(* Logix 5000 AddOnInstructionDefinition export Banner_Q2X_Param_v4; software revision 33.00; part 3 of 3 *)
(* tags used below, declared in another part *)
   Q2X : Banner_Q2X_v4;
   Port_Data : Banner_IOL_Port_v4;
   Port : DINT;
   Local_Control : DINT;
   Command_Being_Processed : BOOL;
   Update_Archive : BOOL;
   Index_Write_Inprocess : INT;
   Inprocess_Index : DINT;
(* Banner_Q2X_Param_v4, continued *)

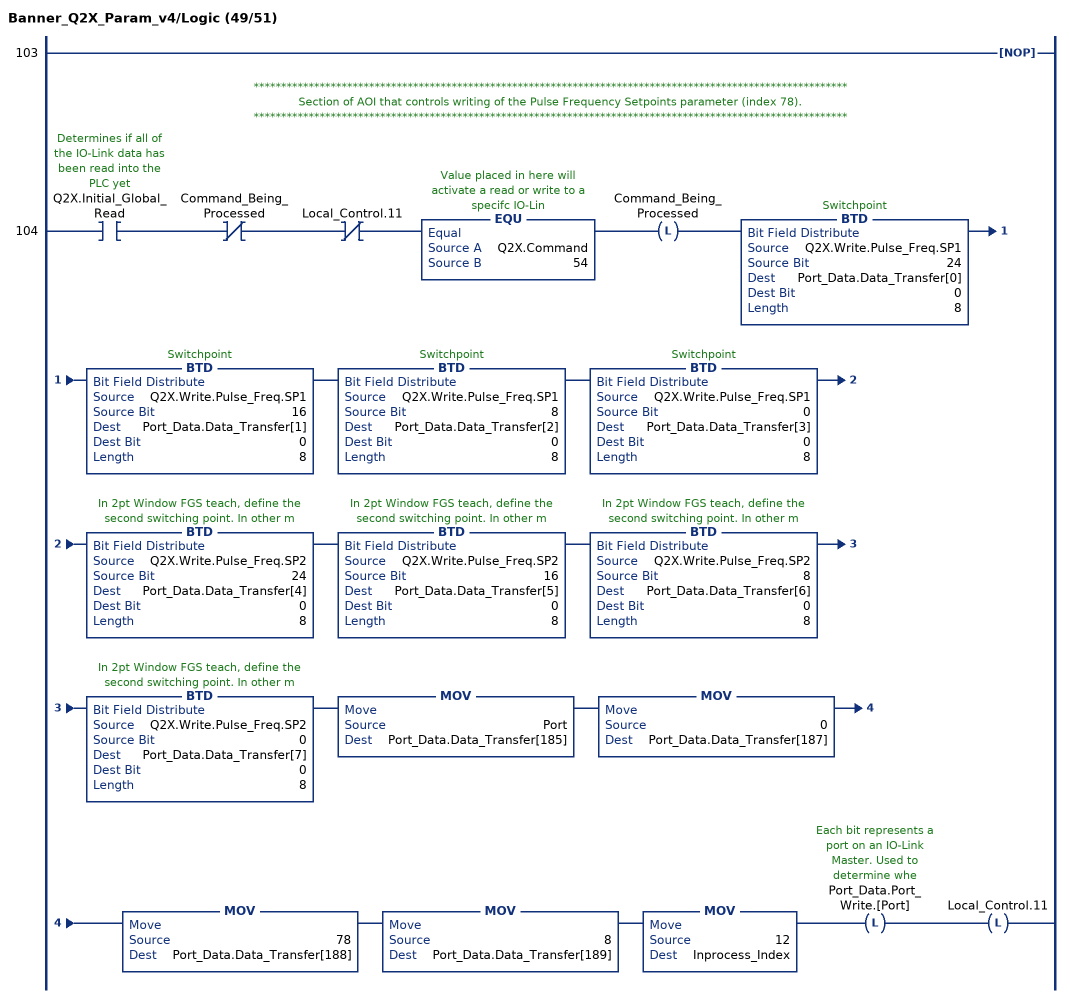
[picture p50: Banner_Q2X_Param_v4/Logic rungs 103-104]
   103: NOP();
   // ************************************************************************************************************
   // Section of AOI that controls writing of the Pulse Frequency Setpoints parameter (index 78).
   // ************************************************************************************************************
   104: XIC(Q2X.Initial_Global_Read)XIO(Command_Being_Processed)XIO(Local_Control.11)EQU(Q2X.Command,54)OTL(Command_Being_Processed)BTD(Q2X.Write.Pulse_Freq.SP1,24,Port_Data.Data_Transfer[0],0,8)BTD(Q2X.Write.Pulse_Freq.SP1,16,Port_Data.Data_Transfer[1],0,8)BTD(Q2X.Write.Pulse_Freq.SP1,8,Port_Data.Data_Transfer[2],0,8)BTD(Q2X.Write.Pulse_Freq.SP1,0,Port_Data.Data_Transfer[3],0,8)BTD(Q2X.Write.Pulse_Freq.SP2,24,Port_Data.Data_Transfer[4],0,8)BTD(Q2X.Write.Pulse_Freq.SP2,16,Port_Data.Data_Transfer[5],0,8)BTD(Q2X.Write.Pulse_Freq.SP2,8,Port_Data.Data_Transfer[6],0,8)BTD(Q2X.Write.Pulse_Freq.SP2,0,Port_Data.Data_Transfer[7],0,8)MOV(Port,Port_Data.Data_Transfer[185])MOV(0,Port_Data.Data_Transfer[187])MOV(78,Port_Data.Data_Transfer[188])MOV(8,Port_Data.Data_Transfer[189])MOV(12,Inprocess_Index)OTL(Port_Data.Port_Write.[Port])OTL(Local_Control.11);
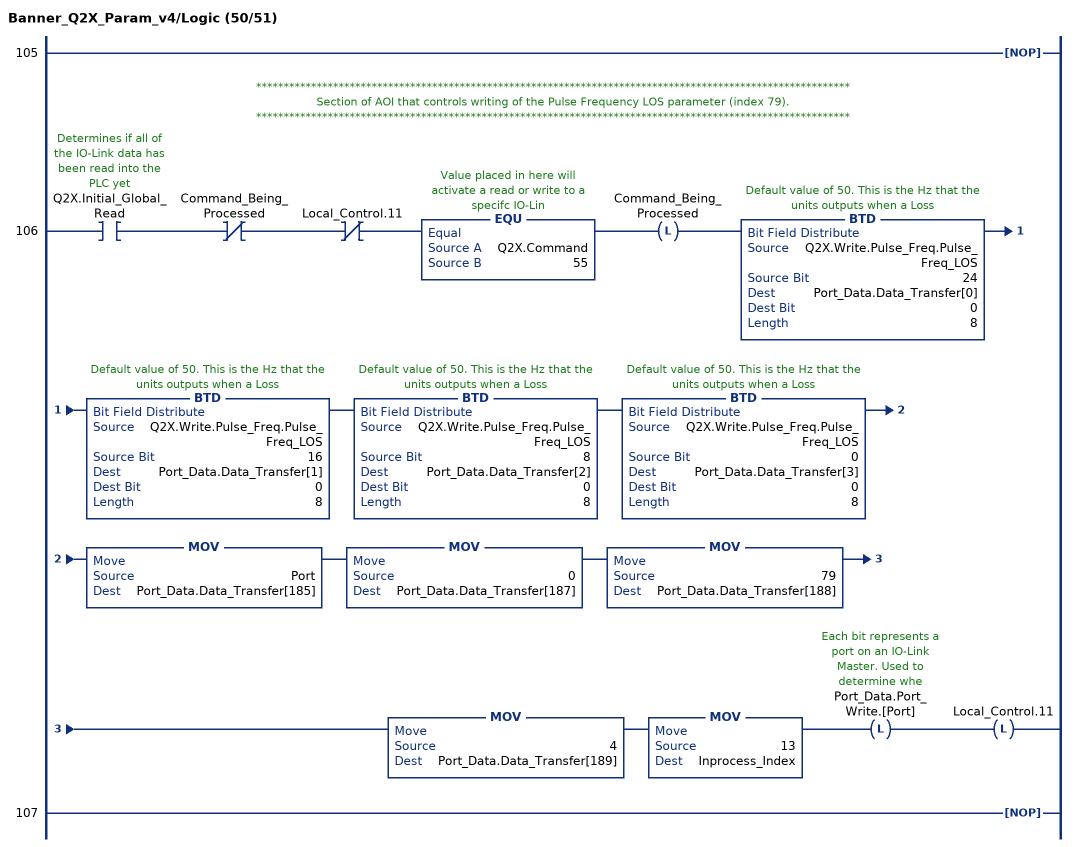
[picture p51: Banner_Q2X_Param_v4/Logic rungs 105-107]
   105: NOP();
   // ************************************************************************************************************
   // Section of AOI that controls writing of the Pulse Frequency LOS parameter (index 79).
   // ************************************************************************************************************
   106: XIC(Q2X.Initial_Global_Read)XIO(Command_Being_Processed)XIO(Local_Control.11)EQU(Q2X.Command,55)OTL(Command_Being_Processed)BTD(Q2X.Write.Pulse_Freq.Pulse_Freq_LOS,24,Port_Data.Data_Transfer[0],0,8)BTD(Q2X.Write.Pulse_Freq.Pulse_Freq_LOS,16,Port_Data.Data_Transfer[1],0,8)BTD(Q2X.Write.Pulse_Freq.Pulse_Freq_LOS,8,Port_Data.Data_Transfer[2],0,8)BTD(Q2X.Write.Pulse_Freq.Pulse_Freq_LOS,0,Port_Data.Data_Transfer[3],0,8)MOV(Port,Port_Data.Data_Transfer[185])MOV(0,Port_Data.Data_Transfer[187])MOV(79,Port_Data.Data_Transfer[188])MOV(4,Port_Data.Data_Transfer[189])MOV(13,Inprocess_Index)OTL(Port_Data.Port_Write.[Port])OTL(Local_Control.11);
   107: NOP();
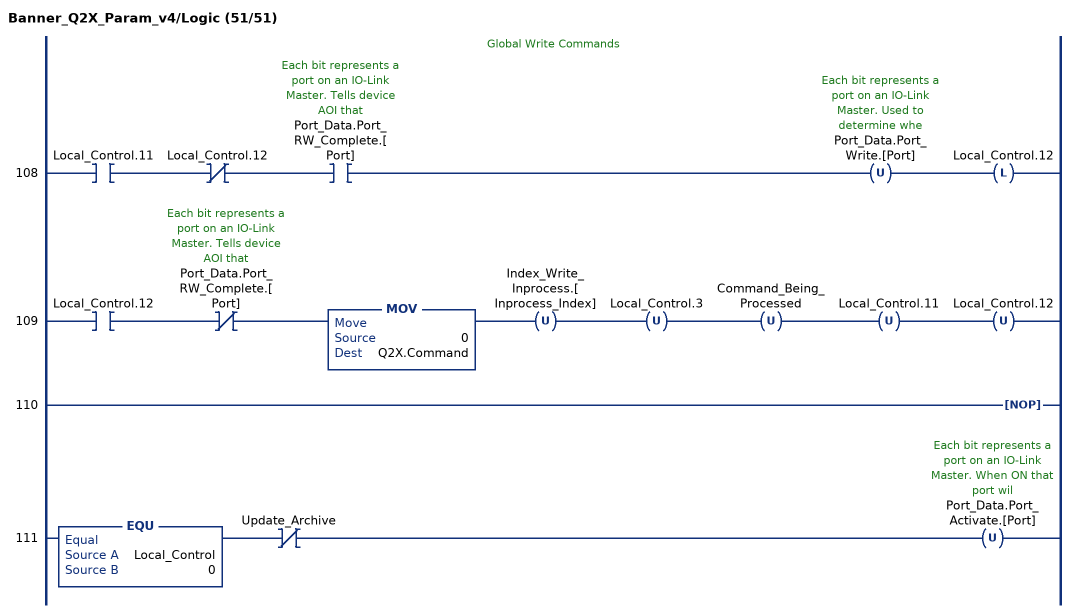
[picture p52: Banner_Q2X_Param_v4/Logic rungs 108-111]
   // Global Write Commands
   108: XIC(Local_Control.11)XIO(Local_Control.12)XIC(Port_Data.Port_RW_Complete.[Port])OTU(Port_Data.Port_Write.[Port])OTL(Local_Control.12);
   109: XIC(Local_Control.12)XIO(Port_Data.Port_RW_Complete.[Port])MOV(0,Q2X.Command)OTU(Index_Write_Inprocess.[Inprocess_Index])OTU(Local_Control.3)OTU(Command_Being_Processed)OTU(Local_Control.11)OTU(Local_Control.12);
   110: NOP();
   111: EQU(Local_Control,0)XIO(Update_Archive)OTU(Port_Data.Port_Activate.[Port]);
END_ROUTINE
END_ADD_ON_INSTRUCTION
